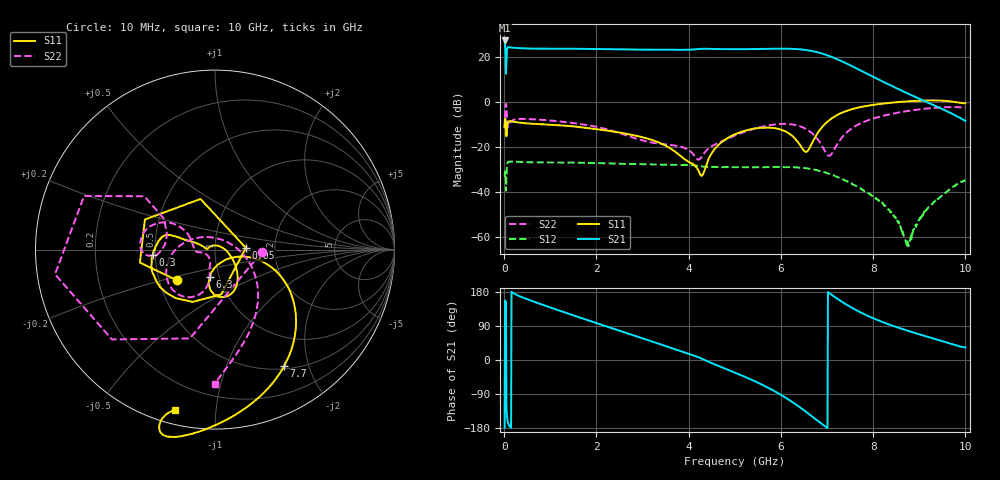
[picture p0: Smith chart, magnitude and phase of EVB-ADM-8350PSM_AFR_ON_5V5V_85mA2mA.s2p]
!Keysight Technologies,N5247B,US58420632,A.15.75.19
!Date: Monday, January 30, 2023 13:22:26
!Correction: S11(C  2-Port  )
!S21(C  2-Port  )
!S12(C  2-Port  )
!S22(C  2-Port  )
!S2P File: Measurements: S11, S21, S12, S22:
# Hz S  dB  R 50
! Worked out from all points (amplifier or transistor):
!   1000 points, 10 MHz to 10 GHz, reference 50 ohm
!   highest |S21| = 27.2 dB at 10 MHz (marker M1)
!   |S21| within 3 dB of that: 88.09 MHz to 111.9 MHz (23.86 MHz wide, 23.9 % of centre)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
!   unconditionally stable (mu >= 1): 33.44 MHz to 872.2 MHz; 2.23 GHz to 8.6 GHz; 9.829 GHz to end of sweep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
!   at 1.67 GHz: K = 0.98, MSG = 25.2 dB, |S12| = -27.0 dB
!   at 5.01 GHz: K = 1.13, MAG = 23.9 dB, |S12| = -28.9 dB
!   at 10 GHz: K = 4.16, MAG = 4.0 dB, |S12| = -34.8 dB
!   S11 on the Smith chart (normalised r, x): 10 MHz: 0.62, -0.23; 50 MHz: 1.42, +0.03; 300 MHz: 0.48, -0.04; 6.3 GHz: 0.90, -0.28; 7.7 GHz: 0.54, -1.62; 10 GHz: 0.07, -0.78
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1e7  -11.29 -141.3  27.16 -179.7  -33.22 74.5  -11.66 -3.2
5e7  -15.28 3.2  18.18 -129.5  -33.31 82.1  -2.07 157.7
8e7  -9.16 -129.1  24.09 -163.5  -26.84 37.9  -11.06 162.8
1e8  -8.64 -145.6  24.19 -171.0  -26.49 26.8  -10.59 -179.9
1.3e8  -8.66 -156.2  24.08 -176.3  -26.46 17.9  -9.25 -175.2
3e8  -9.14 -174.7  23.79 170.2  -26.56 -0.5  -7.65 178.9
1.02e9  -10.20 168.5  23.51 137.8  -26.83 -29.8  -8.29 160.3
1.68e9  -11.31 162.5  23.45 110.5  -27.00 -51.5  -9.93 151.5
2.47e9  -13.52 161.5  23.21 78.5  -27.44 -77.0  -13.65 147.6
3.34e9  -17.91 160.8  23.05 43.3  -27.75 -106.5  -18.49 174.1
4.32e9  -31.56 56.7  23.49 1.4  -28.71 -145.6  -23.26 -113.6
5.01e9  -14.32 -49.1  23.28 -33.5  -28.93 -169.9  -14.89 -100.8
5.42e9  -11.85 -66.5  23.35 -55.2  -28.99 172.8  -11.91 -107.4
5.79e9  -11.50 -83.4  23.47 -77.5  -28.96 155.4  -10.20 -121.1
6.06e9  -12.75 -95.6  23.52 -96.3  -28.89 140.8  -9.75 -135.1
6.3e9  -16.15 -101.1  23.39 -115.3  -29.04 125.6  -10.20 -151.1
6.67e9  -18.42 -20.4  22.50 -148.3  -29.81 99.0  -13.82 175.6
6.9e9  -11.05 -14.6  21.32 -169.9  -30.91 81.4  -19.80 137.9
7.18e9  -6.31 -29.6  19.21 165.2  -32.92 62.2  -20.22 16.5
7.7e9  -2.44 -59.3  14.19 127.3  -38.15 32.7  -9.78 -42.6
8.34e9  -0.52 -85.1  7.65 94.0  -47.67 4.4  -5.61 -70.7
1e10  -0.71 -103.8  -8.46 33.1  -34.80 118.1  -2.53 -90.1
